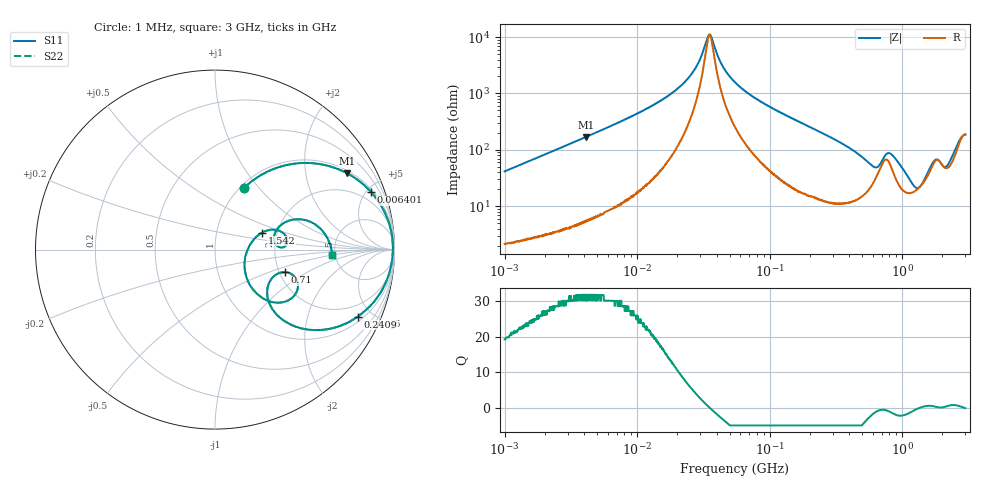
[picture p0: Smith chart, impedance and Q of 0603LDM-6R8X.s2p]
!s-Parameter Generated by FASTRON Sdn. Bhd.
!FASTRON P/N : 0603LDM-6R8X
!Keysight Technologies: E4991B_MY54100416_A.01.15
!Date: Thu Nov 27 16:25:37 2025
!Version  :Rev00  Thu Nov 27 16:25:37 2025
!Data & Calibration Information:
!Freq  S11  S21  S12  S22
!PortZ  Port1:50+j0  Port2:50+j0
!When reading reference impedance value at option line is always used.
! Remarks : This data is being provided solely for informational purposes.
# Hz S dB R 50
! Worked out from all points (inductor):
!   1601 points, 1 MHz to 3 GHz, reference 50 ohm
!   read as one part in series: L = 6.58 uH near 1.041 MHz
!   highest Q = 31.8 at 4.121 MHz (marker M1), where L = 6.56 uH
!   self-resonance near 35.26 MHz
!   S11 on the Smith chart (normalised r, x): 1 MHz: 1.04, +0.83; 6.401 MHz: 1.18, +5.36; 240.9 MHz: 1.26, -4.13; 710 MHz: 2.15, -0.65; 1.542 GHz: 1.67, +0.34; 3 GHz: 4.72, -0.50
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1000000  -8.46 64.9  -0.85 -22.1  -0.85 -22.1  -8.46 64.9
3804036  -1.61 32.0  -5.51 -56.2  -5.51 -56.2  -1.61 32.0
4121125  -1.41 30.0  -6.02 -58.2  -6.02 -58.2  -1.41 30.0
6401142  -0.66 20.2  -9.23 -67.9  -9.23 -67.9  -0.66 20.2
1.447069e7  -0.15 8.0  -17.10 -78.8  -17.10 -78.8  -0.15 8.0
2.509235e7  -0.08 2.7  -26.30 -77.6  -26.30 -77.6  -0.08 2.7
3.508696e7  -0.08 0.0  -41.00 -4.3  -41.00 -4.3  -0.08 0.0
4.394807e7  -0.09 -1.7  -30.00 70.9  -30.00 70.9  -0.09 -1.7
5.504702e7  -0.10 -3.6  -24.00 77.3  -24.00 77.3  -0.10 -3.6
2.083556e8  -0.85 -21.7  -8.61 64.8  -8.61 64.8  -0.85 -21.7
2.408952e8  -1.12 -25.1  -7.44 61.3  -7.44 61.3  -1.12 -25.1
4.457915e8  -3.99 -43.2  -3.20 38.7  -3.20 38.7  -3.99 -43.2
5.959055e8  -8.14 -41.8  -2.45 20.3  -2.45 20.3  -8.14 -41.8
7.099691e8  -7.73 -17.8  -4.12 11.7  -4.12 11.7  -7.73 -17.8
7.925923e8  -5.90 -24.4  -4.77 21.3  -4.77 21.3  -5.90 -24.4
9.585869e8  -7.60 -43.6  -2.44 22.4  -2.44 22.4  -7.60 -43.6
1.281378e9  -15.10 -19.0  -1.56 3.9  -1.56 3.9  -15.10 -19.0
1.542004e9  -11.10 19.8  -2.56 -7.3  -2.56 -7.3  -11.10 19.8
1.75626e9  -7.99 11.8  -4.22 -7.7  -4.22 -7.7  -7.99 11.8
1.970482e9  -8.77 1.9  -3.93 -1.1  -3.93 -1.1  -8.77 1.9
2.480502e9  -5.80 19.1  -5.31 -18.0  -5.31 -18.0  -5.80 19.1
3e9  -3.69 -2.7  -9.17 5.0  -9.17 5.0  -3.69 -2.7
